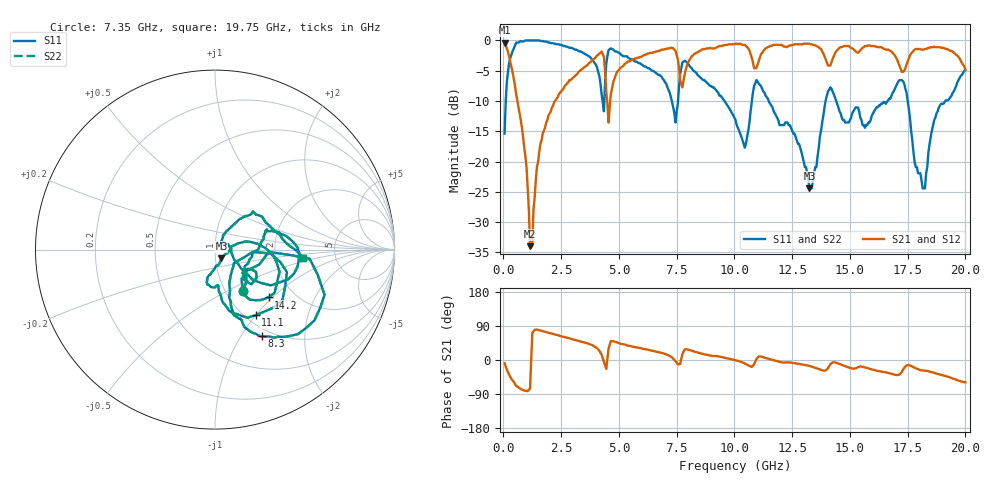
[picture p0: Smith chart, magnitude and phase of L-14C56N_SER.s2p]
# MHZ S MA R 50
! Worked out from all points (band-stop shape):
!   400 points, 50 MHz to 20 GHz, reference 50 ohm
!   highest |S21| = -0.35 dB at 50 MHz (marker M1); lowest = -34.0 dB at 1.15 GHz (marker M2)
!   |S21| within 3 dB of the highest: 11.06 GHz to 13.98 GHz (2.915 GHz wide, 23.3 % of centre); 14.22 GHz to 17.06 GHz (2.838 GHz wide, 18.1 % of centre)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
!   lowest |S11| = -24.4 dB at 13.25 GHz (marker M3), VSWR 1.13, Z = 53.4 - j5.18 ohm
!   |S11| at or under -10 dB: 11.48 GHz to 13.95 GHz (2.461 GHz wide, 19.4 % of centre); 14.41 GHz to 16.63 GHz (2.222 GHz wide, 14.3 % of centre); 17.5 GHz to 19.13 GHz (1.628 GHz wide, 8.89 % of centre)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
!   |S22| runs from -24.4 to 0.0 dB; largest |S21 - S12| = 0
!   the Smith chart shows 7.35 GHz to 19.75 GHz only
!   S11 on the Smith chart (normalised r, x): 7.35 GHz: 1.20, -0.61; 8.3 GHz: 0.90, -1.24; 11.1 GHz: 1.11, -1.00; 14.2 GHz: 1.49, -0.95; 19.75 GHz: 2.88, -0.34
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50  0.17 73.1  0.96 -8.5  0.96 -8.5  0.17 73.1
300  0.72 40.9  0.66 -44.9  0.66 -44.9  0.72 40.9
1150  1 4.5  0.02 -75.9  0.02 -75.9  1 4.5
1700  0.99 -9.1  0.17 76.3  0.17 76.3  0.99 -9.1
3400  0.8 -42.4  0.58 48.2  0.58 48.2  0.8 -42.4
4250  0.36 -59.7  0.81 14.1  0.81 14.1  0.36 -59.7
4450  0.64 -0.3  0.38 -23.4  0.38 -23.4  0.64 -0.3
4900  0.81 -46.2  0.54 46.7  0.54 46.7  0.81 -46.2
6700  0.52 -63.3  0.82 21.0  0.82 21.0  0.52 -63.3
7350  0.28 -56.4  0.86 3.8  0.86 3.8  0.28 -56.4
7750  0.66 -22.4  0.41 16.4  0.41 16.4  0.66 -22.4
8300  0.55 -61.5  0.78 21.7  0.78 21.7  0.55 -61.5
10050  0.22 -68.5  0.94 -0.6  0.94 -0.6  0.22 -68.5
11100  0.43 -58.3  0.72 9.2  0.72 9.2  0.43 -58.3
13250  0.06 -53.6  0.94 -15.5  0.94 -15.5  0.06 -53.6
13350  0.06 -29.9  0.93 -17.5  0.93 -17.5  0.06 -29.9
14200  0.4 -41.8  0.66 -8.8  0.66 -8.8  0.4 -41.8
16700  0.33 18.5  0.83 -34.8  0.83 -34.8  0.33 18.5
17350  0.44 -22.2  0.56 -20.8  0.56 -20.8  0.44 -22.2
18250  0.06 53.1  0.85 -28.2  0.85 -28.2  0.06 53.1
19750  0.49 -5.2  0.71 -55.4  0.71 -55.4  0.49 -5.2
20000  0.57 -16.1  0.57 -58.8  0.57 -58.8  0.57 -16.1
